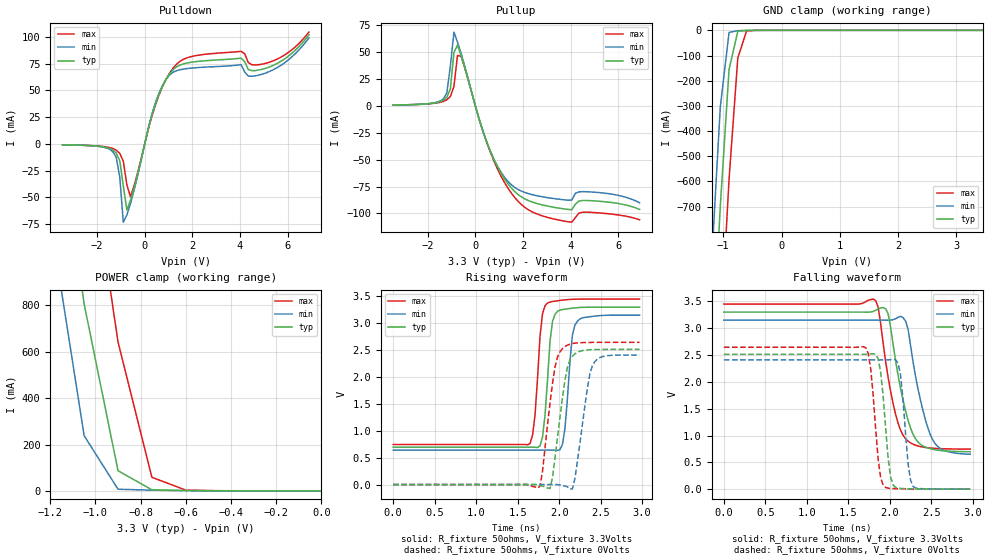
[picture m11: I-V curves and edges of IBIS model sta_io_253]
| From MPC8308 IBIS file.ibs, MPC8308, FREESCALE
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[Model]   sta_io_253   |
Model_type   I/O
Vinl = 0.8
Vinh = 2
Vmeas = 1.65
Cref = 5E-11
Rref = 50
Vref = 0
| variable   typ   min   max
C_comp   494.81f   465.60f   523.27f
[Model Spec]
| subparameter   typ   min   max
S_overshoot_high  3.300   3.135   3.465
S_overshoot_low   -200.00m  -100.00m  -300.00m
D_overshoot_high  4.000   4.000   4.000
D_overshoot_low   -1.000   -1.000   -1.000
D_overshoot_time  1.000n   1.000n   1.000n
| variable   typ   min   max
[Temperature Range]   55.0   110.0   0.0
| variable   typ   min   max
[Pullup Reference]   3.300V   3.150V   3.450V
| variable   typ   min   max
[Pulldown Reference]   0.000V   0.000V   0.000V
| variable   typ   min   max
[POWER_Clamp_Reference]   3.300V   3.150V   3.450V
| variable   typ   min   max
[GND_Clamp_Reference]   0.000V   0.000V   0.000V
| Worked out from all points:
|   slope of the pulldown table from 0 to 0.495 V, typ, clamps not added: 12.4 ohm
|   slope of the pullup table from 0 to 0.495 V, typ, clamps not added: 14.5 ohm
|   GND clamp passes 1 mA (typ) near -0.62 V on its own axis
|   POWER clamp passes 1 mA (typ) near -0.51 V on its own axis
|   rising waveform, R_fixture 50ohms, V_fixture 3.3Volts: 20-80 % time 74.9ps typ, 76.6ps min, 71.7ps max; typ from 0.695 V to 3.3 V
|   rising waveform, R_fixture 50ohms, V_fixture 0Volts: 20-80 % time 128ps typ, 131ps min, 124ps max; typ from 0 V to 2.51 V
|   falling waveform, R_fixture 50ohms, V_fixture 3.3Volts: 20-80 % time 201ps typ, 204ps min, 185ps max; typ from 3.3 V to 0.698 V
|   falling waveform, R_fixture 50ohms, V_fixture 0Volts: 20-80 % time 84.8ps typ, 77.1ps min, 84.3ps max; typ from 2.51 V to 0 V
[Pulldown]
| pulldown in the table = pulldown subtract gnd_clamp
|Voltage   I(typ)   I(min)   I(max)
-3.45V    -872.5uA   -841.3uA   -848.6uA
-1.35V    -5.535mA   -6.95mA    -4.235mA
-1.05V    -15.56mA   -30.43mA   -8.792mA
-900mV    -39.07mA   -73.08mA   -16.14mA
-750mV    -61.82mA   -66.44mA   -38.16mA
-600mV    -52.74mA   -55.84mA   -49.36mA
300mV     26.56mA    27.73mA    25.65mA
1.05V     65.58mA    64.47mA    66.21mA
2.85V     78.08mA    71.99mA    84.3mA
4.05V     80.02mA    73.94mA    86.37mA
4.8V      68.94mA    64.22mA    73.92mA
6.9V      101.8mA    98.94mA    104.3mA
[Pullup]
| pullup in the table = pullup subtract power_clamp
|Voltage   I(typ)   I(min)   I(max)
-3.45V    852.6uA    819.4uA    863.3uA
-1.35V    5.175mA    6.43mA     4.157mA
-1.2V     7.937mA    11.75mA    5.684mA
-1.05V    15.86mA    37.13mA    8.855mA
-900mV    49.77mA    68.77mA    18.16mA
-750mV    56.61mA    59.5mA     47.07mA
-600mV    46.84mA    49.13mA    46.26mA
450mV     -31.6mA    -32.16mA   -32.23mA
1.5V      -76.09mA   -73.12mA   -80.8mA
3.45V     -94.9mA    -86.63mA   -106mA
4.65V     -87.99mA   -79.84mA   -98.86mA
6.9V      -96.28mA   -90.1mA    -105.9mA
[GND_clamp]
|Voltage   I(typ)   I(min)   I(max)
-3.45V    -12.31A    -11.88A    -12.85A
-1.2V     -1.358A    -924.9mA   -1.906A
-1.05V    -698.5mA   -303.5mA   -1.226A
-900mV    -155.7mA   -8.533mA   -591.6mA
-750mV    -3.954mA   -1.306mA   -110.3mA
-600mV    -606.2uA   -198.8uA   -3.05mA
-300mV    -1.971uA   -109.9nA   -16.38uA
3.45V     171.4nA    873.4nA    35.1nA
[POWER_clamp]
|Voltage   I(typ)   I(min)   I(max)
-3.3V     18.63A     17.95A     19.5A
-1.2V     1.853A     1.171A     2.731A
-1.05V    806.1mA    238.2mA    1.631A
-900mV    87.08mA    7.341mA    642.4mA
-750mV    4.847mA    3.182mA    58.69mA
-600mV    1.868mA    967.7uA    3.546mA
0V        962.3pA    16.62pA    35.1nA
[Ramp]
|Voltage   I(typ)   I(min)   I(max)
dV/dt_f   1.61/204.357p 1.55/208.211p 1.68/187.372p
dV/dt_r   1.56/130.543p 1.51/134.827p 1.63/125.396p
R_load=50ohms
| R_load was connected to ground for Ramp_up test and power for Ramp_dn test
[Rising_Waveform]
R_fixture=50ohms
V_fixture=3.3Volts
V_fixture_min=3.15Volts
V_fixture_max=3.45Volts
|C_fixture=1E-15f
|L_fixture=1E-15h
|C_dut=1E-15fh
|R_dut=0.001ohm
|L_dut=1E-12h
|time   V(typ)   V(min)   V(max)
0s        695mV      642mV      745mV
1.65ns    696mV      642mV      765mV
1.71ns    693mV      642mV      1.303V
1.77ns    722mV      642mV      2.765V
1.83ns    1.29V      642mV      3.325V
1.92ns    3.034V     641mV      3.404V
2.01ns    3.245V     648mV      3.425V
2.07ns    3.262V     1.042V     3.436V
2.19ns    3.286V     2.963V     3.447V
2.97ns    3.3V       3.15V      3.45V
[Rising_Waveform]
R_fixture=50ohms
V_fixture=0Volts
|C_fixture=1E-15f
|L_fixture=1E-15h
|C_dut=1E-15fh
|R_dut=0.001ohm
|L_dut=1E-12h
|time   V(typ)   V(min)   V(max)
0s        0V         0V         0V
1.74ns    -4mV       0V         -67mV
1.8ns     -31mV      0V         254mV
1.89ns    -73mV      0V         1.516V
1.98ns    875mV      -1mV       2.37V
2.07ns    1.938V     -28mV      2.568V
2.16ns    2.388V     -79mV      2.622V
2.34ns    2.504V     1.787V     2.643V
2.4ns     2.51V      2.206V     2.644V
2.97ns    2.514V     2.409V     2.645V
[Falling_Waveform]
R_fixture=50ohms
V_fixture=3.3Volts
V_fixture_min=3.15Volts
V_fixture_max=3.45Volts
|C_fixture=1E-15f
|L_fixture=1E-15h
|C_dut=1E-15fh
|R_dut=0.001ohm
|L_dut=1E-12h
|time   V(typ)   V(min)   V(max)
0s        3.3V       3.15V      3.45V
1.83ns    3.333V     3.15V      3.515V
1.86ns    3.361V     3.15V      3.391V
1.98ns    3.267V     3.148V     2.084V
2.13ns    1.878V     3.222V     1.1V
2.22ns    1.286V     2.987V     895mV
2.28ns    1.024V     2.379V     838mV
2.4ns     806mV      1.466V     785mV
2.52ns    742mV      913mV      763mV
2.97ns    698mV      651mV      746mV
[Falling_Waveform]
R_fixture=50ohms
V_fixture=0Volts
|C_fixture=1E-15f
|L_fixture=1E-15h
|C_dut=1E-15fh
|R_dut=0.001ohm
|L_dut=1E-12h
|time   V(typ)   V(min)   V(max)
0s        2.514V     2.409V     2.645V
1.71ns    2.513V     2.409V     2.636V
1.83ns    2.512V     2.409V     1.119V
1.92ns    1.735V     2.408V     71mV
2.01ns    227mV      2.414V     14mV
2.07ns    32mV       2.412V     9mV
2.13ns    14mV       2.127V     7mV
2.22ns    7mV        483mV      4mV
2.28ns    5mV        52mV       3mV
2.97ns    0V         0V         0V
